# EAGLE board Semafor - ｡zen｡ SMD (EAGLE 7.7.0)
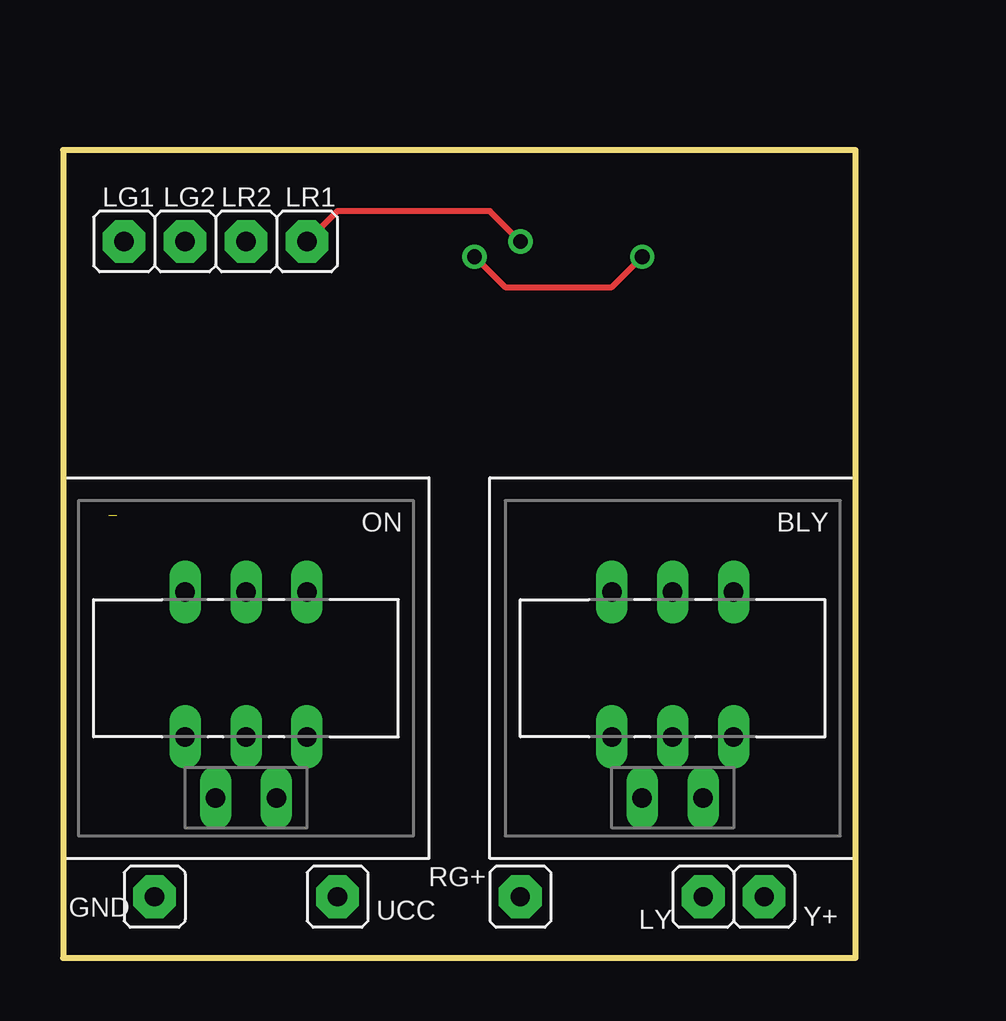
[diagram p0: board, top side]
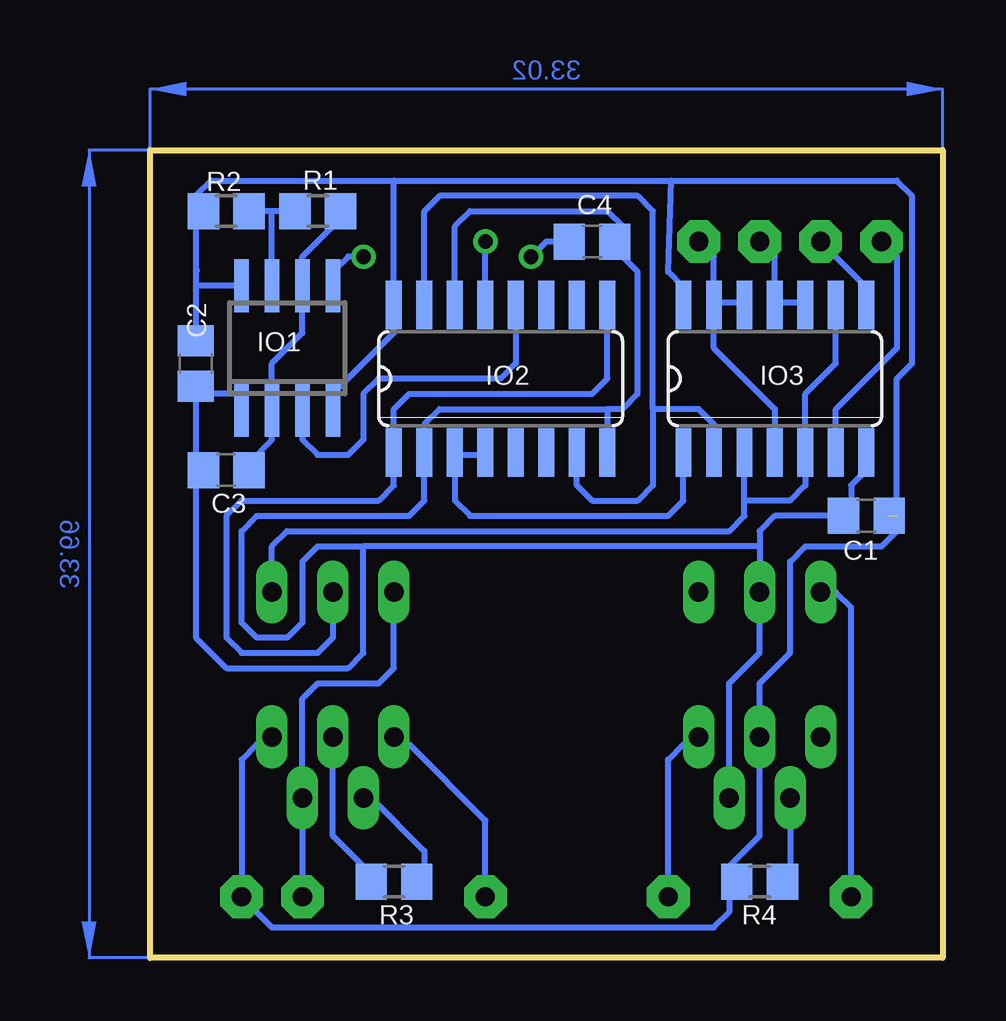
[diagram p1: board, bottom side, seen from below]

Size 33.02 x 33.66 mm. Coordinates in mm from the lower left corner, seen from the top.
Outline: 0,0 33.02,0 33.02,33.66 0,33.66 0,0
Copper layers (1*16): Top 0.035mm / dielectric 1.5mm / Bottom 0.035mm
Design rules "default": minimum track width 10mil, minimum drill 24mil, track to track 8mil, track to pad 8mil, pad to pad 8mil, via to via 8mil, smd to smd 8mil, copper to edge 40mil, drill to drill 8mil, minimum pad ring 10mil, minimum via ring 8mil, stop-mask expansion 4mil, vias tented up to drill 0mil, thermal gap 10mil

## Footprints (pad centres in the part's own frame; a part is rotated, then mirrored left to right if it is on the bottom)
P-0S?B = drill 0.813 pad 1.27 long: 1 2.54,-3.175; 2 0,-3.175; 3 -2.54,-3.175; 4 -2.54,2.857; 5 0,2.857; 6 2.54,2.857; A1 1.27,5.397; K1 -1.27,5.397
C0805 = smd 1.3 x 1.5: 1 -0.95,0; 2 0.95,0
S1G1_JUM = drill 0.8 pad 1.778 octagon: 1 0,0
SO08 = smd 0.6 x 2.2: 1 -1.905,-2.6; 2 -0.635,-2.6; 3 0.635,-2.6; 4 1.905,-2.6; 5 1.905,2.6; 6 0.635,2.6; 7 -0.635,2.6; 8 -1.905,2.6
SO16 = smd 0.66 x 2.032: 1 -4.445,-3.073; 2 -3.175,-3.073; 3 -1.905,-3.073; 4 -0.635,-3.073; 5 0.635,-3.073; 6 1.905,-3.073; 7 3.175,-3.073; 8 4.445,-3.073; 9 4.445,3.073; 10 3.175,3.073; 11 1.905,3.073; 12 0.635,3.073; 13 -0.635,3.073; 14 -1.905,3.073; 15 -3.175,3.073; 16 -4.445,3.073
SO14 = smd 0.66 x 2.032: 1 -3.81,-3.073; 2 -2.54,-3.073; 3 -1.27,-3.073; 4 0,-3.073; 5 1.27,-3.073; 6 2.54,-3.073; 7 3.81,-3.073; 8 3.81,3.073; 9 2.54,3.073; 10 1.27,3.073; 11 0,3.073; 12 -1.27,3.073; 13 -2.54,3.073; 14 -3.81,3.073
R0805 = smd 1.3 x 1.5: 1 -0.95,0; 2 0.95,0

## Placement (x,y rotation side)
BLY  [P-0S?B]  25.4,12.06 180 top
C1  100n  [C0805]  3.17,18.41 180 bottom
C2  100n  [C0805]  31.11,24.77 270 bottom
C3  1u  [C0805]  29.84,20.32 180 bottom
C4  10n  [C0805]  14.61,29.84 0 bottom
GND  [S1G1_JUM]  3.81,2.54 0 top
IO1  CMOS555  [SO08]  27.3,25.4 0 bottom
IO2  74HCT390  [SO16]  18.41,24.13 0 bottom
IO3  74HCT00  [SO14]  6.99,24.13 0 bottom
LG1  [S1G1_JUM]  2.54,29.84 0 top
LG2  [S1G1_JUM]  5.08,29.84 0 top
LR1  [S1G1_JUM]  10.16,29.84 0 top
LR2  [S1G1_JUM]  7.62,29.84 0 top
LY  [S1G1_JUM]  26.67,2.54 0 top
ON  [P-0S?B]  7.62,12.06 180 top
R1  100k  [R0805]  26.04,31.11 0 bottom
R2  100k  [R0805]  29.84,31.11 180 bottom
R3  680R  [R0805]  22.86,3.17 0 bottom
R4  680R  [R0805]  7.62,3.17 0 bottom
RG+  [S1G1_JUM]  19.05,2.54 0 top
UCC  [S1G1_JUM]  11.43,2.54 0 top
Y+  [S1G1_JUM]  29.21,2.54 0 top

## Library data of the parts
BLY ON = #PaJa_prepinace
C1-C4 R1-R4 = rcl
GND LG1 LG2 LR1 LR2 LY RG+ UCC Y+ = #PaJa_konektory
IO1 = #PaJa_31
IO2 IO3 = 74xx-eu

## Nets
N$1: IO2.13 IO3.4 IO3.12 IO3.13 LR1.1
N$2: IO2.7 IO2.15 IO3.2
N$3: IO2.3 IO2.4 IO3.1
N$4: BLY.3 IO3.3 IO3.5 IO3.9
N$5: IO3.10 IO3.11 LR2.1
N$6: IO3.6 LG1.1
N$7: IO3.8 LG2.1
N$8: BLY.4 C1.1 C2.1 IO1.4 IO1.8 IO2.16 IO3.14 ON.5 R2.2 R4.1 Y+.1
N$9: GND.1 ON.1
N$10: ON.4 UCC.1
N$11: ON.A1 R4.2
N$12: C1.2 C2.2 C3.2 C4.2 IO1.1 IO2.2 IO2.8 IO2.14 IO3.7 ON.2 ON.K1
N$13: BLY.6 RG+.1
N$14: BLY.1 BLY.K1 LY.1
N$15: BLY.A1 R3.2
N$16: BLY.5 R3.1
N$21: BLY.2 IO2.1 IO2.9
N$23: IO1.3 IO2.12
N$24: C4.1 IO1.5
N$25: IO1.7 R1.1 R2.1
N$26: C3.1 IO1.2 IO1.6 R1.2

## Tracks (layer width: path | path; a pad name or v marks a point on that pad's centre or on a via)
N$1  (via drill 0.61)
  Top 0.254: v19.05,29.84 17.78,31.11 11.43,31.11 LR1.1
  Bottom 0.254: 9.53,27.3 IO3.13 9.53,25.4 6.99,22.86 IO3.4 | 9.53,27.3 8.36,27.3 IO3.12 | 9.53,27.3 9.53,29.21 LR1.1 | 19.13,27.13 IO2.13 v19.05,29.84 19.05,27.94 19.13,27.86 19.13,27.13
N$2
  Bottom 0.254: 12.06,22.86 12.06,19.68 12.7,19.05 14.61,19.05 15.24,19.68 IO2.7 | IO3.2 9.53,22.23 10.16,22.86 12.06,22.86 | IO2.15 21.59,31.11 20.95,31.75 12.7,31.75 12.06,31.11 12.06,22.86
N$3
  Bottom 0.254: IO3.1 10.79,19.05 11.43,18.41 19.68,18.41 20.32,19.05 20.32,20.95 | IO2.3 20.32,20.95 | 20.32,20.95 19.15,20.95 IO2.4
N$4
  Bottom 0.254: 8.26,20.95 IO3.3 8.26,19.05 | IO3.9 4.45,24.77 5.71,23.5 IO3.5 5.71,19.68 6.35,19.05 8.26,19.05 | 8.26,19.05 8.26,18.41 8.89,17.78 27.3,17.78 27.94,17.14 BLY.3
N$5
  Bottom 0.254: 5.71,27.3 IO3.10 5.82,27.3 6.88,27.3 IO3.11 6.99,29.21 LR2.1
N$6
  Bottom 0.254: IO3.6 4.45,22.86 1.91,25.4 1.91,29.21 LG1.1
N$7
  Bottom 0.254: LG2.1 3.17,27.94 IO3.8
N$8  (1 unrouted)
  Bottom 0.254: IO1.4 25.4,23.5 22.86,26.04 IO2.16 22.86,32.38 | 31.11,30.48 31.11,28.57 | 31.11,28.57 31.11,27.94 | 31.11,27.94 C2.1 | R2.2 31.11,30.48 | BLY.4 28.26,8.89 28.57,8.89 29.21,8.26 Y+.1 27.94,1.27 9.53,1.27 8.89,1.91 8.89,2.54 R4.1 8.89,2.86 8.89,3.81 7.62,5.08 ON.5 7.62,11.43 6.35,12.7 6.35,16.51 5.71,17.14 2.54,17.14 1.91,17.78 1.91,18.41 | C1.1 2.23,18.73 1.91,19.05 1.91,24.13 1.27,24.77 1.27,31.75 1.91,32.38 11.3,32.38 | 10.79,27.3 10.9,27.3 IO3.14 10.79,27.3 | 10.79,27.3 10.79,27.94 11.43,28.57 11.3,32.38 | 31.11,30.48 31.11,31.75 30.48,32.38 22.86,32.38 | 22.86,32.38 11.3,32.38 | 31.05,28.64 31.11,28.57 | IO1.8 31.05,28 31.11,27.94
N$9
  Bottom 0.254: ON.1 4.45,15.24 3.81,14.61 GND.1
N$10
  Bottom 0.254: UCC.1 11.43,8.26 10.79,8.89 10.48,8.89 ON.4
N$11
  Bottom 0.254: ON.A1 6.35,2.86 R4.2
N$12
  Bottom 0.254: 13.97,22.86 20.95,22.86 21.59,22.23 IO2.2 21.59,19.05 22.23,18.41 28.57,18.41 29.21,17.78 29.21,13.97 28.57,13.34 27.3,13.34 26.67,13.97 26.67,16.51 26.04,17.14 24.13,17.14 | 13.97,22.86 IO2.8 | 3.17,21.59 IO3.7 3.17,20.32 3.81,19.68 3.81,18.73 C1.2 6.99,18.41 7.62,17.78 7.62,17.14 | 24.13,17.14 24.13,12.7 24.77,12.06 29.84,12.06 31.11,13.34 31.11,19.68 30.8,20 C3.2 31.11,20.64 C2.2 30.8,23.5 29.21,23.5 IO1.1 | ON.K1 8.89,11.43 7.62,12.7 ON.2 7.62,17.14 | 13.97,22.86 13.34,22.86 12.7,23.5 12.7,28.57 13.34,29.21 13.34,29.52 C4.2 13.34,30.16 13.34,30.48 13.97,31.11 19.68,31.11 20.32,30.48 IO2.14 | 7.62,17.14 24.13,17.14
N$13
  Bottom 0.254: BLY.6 22.54,8.89 22.23,8.89 19.05,5.71 RG+.1
N$14
  Bottom 0.254: BLY.1 22.86,12.06 23.5,11.43 26.04,11.43 26.67,10.79 BLY.K1 LY.1
N$15
  Bottom 0.254: BLY.A1 23.81,6.67 21.59,4.45 21.59,2.86 R3.2
N$16
  Bottom 0.254: R3.1 24.13,2.54 24.13,3.81 25.4,5.08 BLY.5
N$21
  Bottom 0.254: IO2.9 13.97,24.13 14.61,23.5 22.23,23.5 22.86,22.86 IO2.1 22.86,19.68 23.5,19.05 29.21,19.05 29.84,18.41 29.84,13.34 29.21,12.7 26.04,12.7 25.4,13.34 BLY.2
N$23
  Bottom 0.254: IO2.12 17.78,24.77 18.41,24.13 23.5,24.13 24.13,23.5 24.13,21.59 24.77,20.95 26.04,20.95 26.67,21.59 IO1.3
N$24  (via drill 0.61)
  Top 0.254: v17.14,29.21 18.41,27.94 22.86,27.94 v24.13,29.21
  Bottom 0.254: v24.13,29.21 24.77,29.21 25.4,28.57 IO1.5 | C4.1 16.51,29.84 v17.14,29.21
N$25
  Bottom 0.254: R1.1 27.94,31.11 | 27.94,31.11 R2.1 | IO1.7 27.94,31.11
N$26
  Bottom 0.254: R1.2 25.4,30.8 25.4,30.48 26.67,29.21 IO1.6 26.67,26.04 27.94,24.77 IO1.2 27.94,21.59 28.89,20.64 C3.1
(copper drawn outside any net)
  shapes: Bottom area x2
